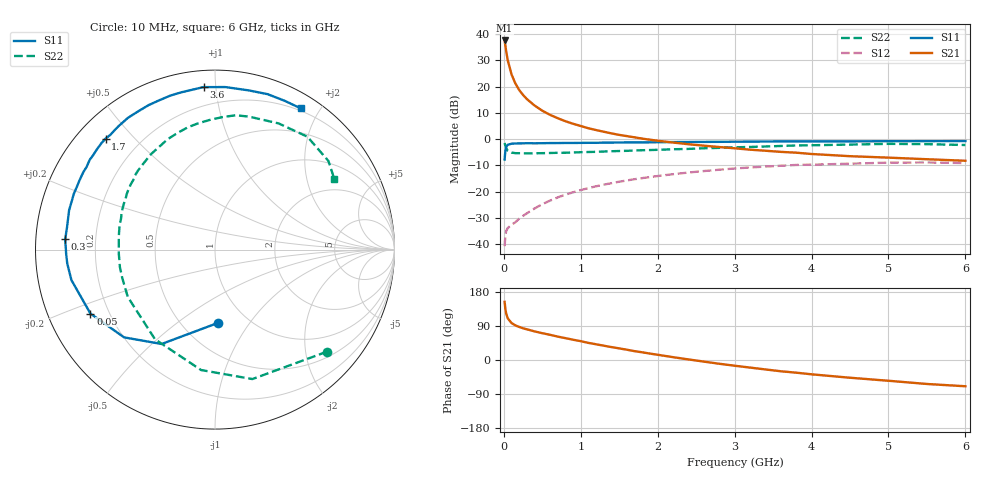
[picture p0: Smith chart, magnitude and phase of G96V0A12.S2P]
! SIEMENS Small Signal Semiconductors
! BFG235
! Si NPN RF Bipolar Junction Transistor in SOT223
! VCE = 6 V  IC = 120 mA
! Common Emitter S-Parameters:  July  1994
# GHz  S  MA  R  50
!  f  S11  S21  S12  S22
! GHz  MAG  ANG  MAG  ANG  MAG  ANG  MAG  ANG
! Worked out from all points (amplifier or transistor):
!   40 points, 10 MHz to 6 GHz, reference 50 ohm
!   highest |S21| = 37.6 dB at 10 MHz (marker M1)
!   |S21| within 3 dB of that: start of sweep to 25.14 MHz
!   unconditionally stable (mu >= 1): 462.5 MHz to 1.424 GHz
!   at 200 MHz: K = 0.79, MSG = 24.5 dB, |S12| = -30.3 dB
!   at 1.5 GHz: K = 0.99, MSG = 8.9 dB, |S12| = -16.2 dB
!   at 6 GHz: K = 0.89, MSG = 0.4 dB, |S12| = -9.1 dB
!   S11 on the Smith chart (normalised r, x): 10 MHz: 0.73, -0.72; 50 MHz: 0.13, -0.24; 300 MHz: 0.09, +0.03; 1.7 GHz: 0.08, +0.42; 3.6 GHz: 0.09, +0.93; 6 GHz: 0.17, +1.76
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0.01  0.4088 -87.7  76.17 153.5  0.0091 63.8  0.8445 -42.3
0.02  0.6042 -119.5  60.81 134.8  0.0144 49.5  0.7507 -73.9
0.03  0.704 -136.0  48.13 123.0  0.0176 42.7  0.6754 -96.6
0.05  0.7802 -152.8  32.3 110.1  0.0201 34.5  0.601 -123.8
0.1  0.8177 -168.0  17.14 97.5  0.0233 35.8  0.5529 -151.5
0.15  0.8268 -174.6  11.53 91.3  0.0261 41.7  0.5404 -163.0
0.2  0.8296 -178.3  8.624 87.2  0.0304 46.4  0.5388 -169.5
0.25  0.8326 178.4  6.95 83.7  0.0344 50.1  0.5361 -174.0
0.3  0.8367 176.1  5.801 81.0  0.0385 52.4  0.5364 -177.7
0.4  0.8337 171.6  4.368 75.5  0.0477 56.1  0.5365 177.1
0.5  0.8367 168.0  3.486 70.7  0.0575 57.3  0.5404 172.8
0.6  0.842 164.9  2.909 66.5  0.0672 57.1  0.5441 168.9
0.8  0.8458 158.5  2.197 57.7  0.0875 56.0  0.5506 162.2
1.1  0.8513 149.4  1.611 45.1  0.1164 51.5  0.5685 153.3
1.4  0.8589 142.2  1.287 34.0  0.1446 45.8  0.5878 145.0
1.7  0.8685 134.6  1.082 23.3  0.1725 39.7  0.608 137.1
2.2  0.8799 123.4  0.862 7.5  0.2146 28.6  0.6409 123.6
3.2  0.8962 102.1  0.63 -20.0  0.288 5.5  0.71 97.5
3.6  0.9077 94.0  0.572 -29.7  0.3108 -4.5  0.7408 86.4
4.5  0.9067 78.1  0.473 -46.8  0.3405 -24.4  0.7872 63.3
5.5  0.9154 64.9  0.414 -63.3  0.3593 -46.5  0.802 38.0
6  0.9204 58.8  0.387 -69.3  0.3496 -54.8  0.7723 30.6
